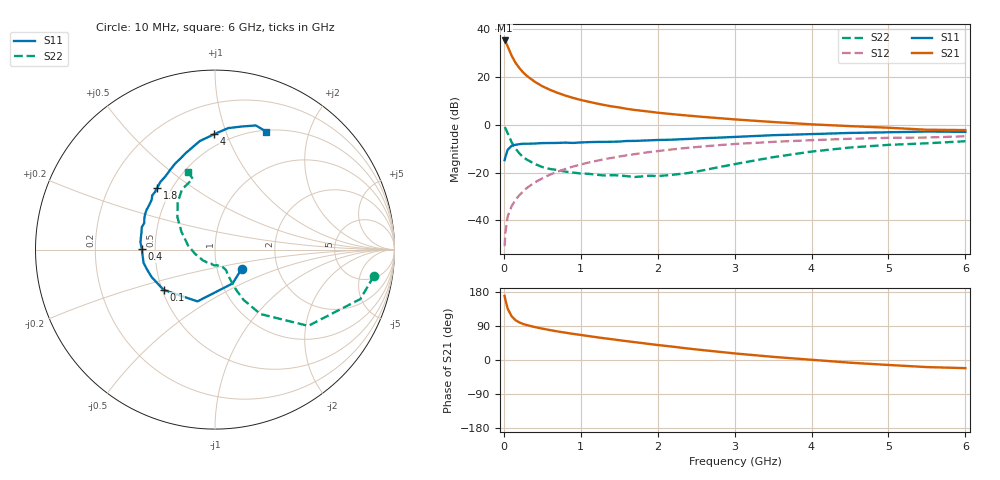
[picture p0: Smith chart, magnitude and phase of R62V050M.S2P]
! SIEMENS Small Signal Semiconductors
! BFR193
! Si NPN RF Bipolar Junction Transistor in SOT23
! VCE = 2 V  IC = 50 mA
! Common Emitter S-Parameters:  May  1996
# GHz  S  MA  R  50
!  f  S11  S21  S12  S22
! GHz  MAG  ANG  MAG  ANG  MAG  ANG  MAG  ANG
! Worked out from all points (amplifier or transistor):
!   36 points, 10 MHz to 6 GHz, reference 50 ohm
!   highest |S21| = 35.4 dB at 10 MHz (marker M1)
!   |S21| within 3 dB of that: start of sweep to 56.81 MHz
!   unconditionally stable (mu >= 1): 337.2 MHz to 1.887 GHz
!   at 250 MHz: K = 0.97, MSG = 24.9 dB, |S12| = -27.9 dB
!   at 1.4 GHz: K = 1.03, MAG = 9.8 dB, |S12| = -13.8 dB
!   at 6 GHz: K = 0.96, MSG = 1.3 dB, |S12| = -4.7 dB
!   S11 on the Smith chart (normalised r, x): 10 MHz: 1.32, -0.29; 100 MHz: 0.51, -0.26; 400 MHz: 0.42, +0.00; 1.8 GHz: 0.42, +0.37; 4 GHz: 0.41, +0.91; 6 GHz: 0.52, +1.40
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0.01  0.1834 -35.1  58.75 169.1  0.0029 80.6  0.8976 -9.4
0.02  0.2126 -62.6  56.13 158.8  0.0056 74.9  0.8551 -18.8
0.05  0.3045 -108.7  44.15 135.6  0.0122 70.7  0.671 -39.3
0.1  0.3637 -141.8  28.49 115.7  0.0198 69.5  0.4392 -54.8
0.15  0.3847 -156.5  20.28 105.3  0.0268 70.2  0.3221 -60.4
0.2  0.3955 -164.2  15.64 99.4  0.0337 72.5  0.2561 -62.2
0.25  0.4046 -169.5  12.63 95.1  0.0405 73.3  0.2136 -62.8
0.3  0.4044 -173.6  10.62 92.0  0.0481 74.6  0.1881 -62.8
0.4  0.4081 179.4  8.069 87.1  0.0623 74.6  0.153 -62.9
0.5  0.4173 174.4  6.475 82.8  0.0763 74.4  0.1315 -61.7
0.6  0.4184 170.7  5.438 78.9  0.0912 73.6  0.1199 -63.1
0.7  0.4209 166.6  4.693 75.3  0.1055 72.8  0.1137 -64.7
0.9  0.4209 159.5  3.685 69.0  0.1348 70.1  0.1006 -68.3
1.1  0.4364 153.2  3.069 63.2  0.1629 67.6  0.0949 -75.0
1.4  0.4454 144.0  2.452 55.0  0.2043 63.2  0.0889 -87.0
1.8  0.4706 133.4  1.977 44.7  0.2582 57.0  0.0839 -109.8
2.2  0.4927 124.1  1.677 35.1  0.3092 50.7  0.0909 -139.3
3.5  0.6106 98.0  1.152 8.3  0.4427 29.6  0.2114 152.1
4  0.6435 90.3  1.03 0.6  0.4801 22.5  0.2774 139.1
4.5  0.681 83.8  0.946 -7.1  0.5131 15.4  0.3368 128.1
5.5  0.7282 71.8  0.794 -18.7  0.5459 1.6  0.4134 107.4
6  0.7165 66.4  0.781 -21.5  0.5794 -2.4  0.4563 109.2
